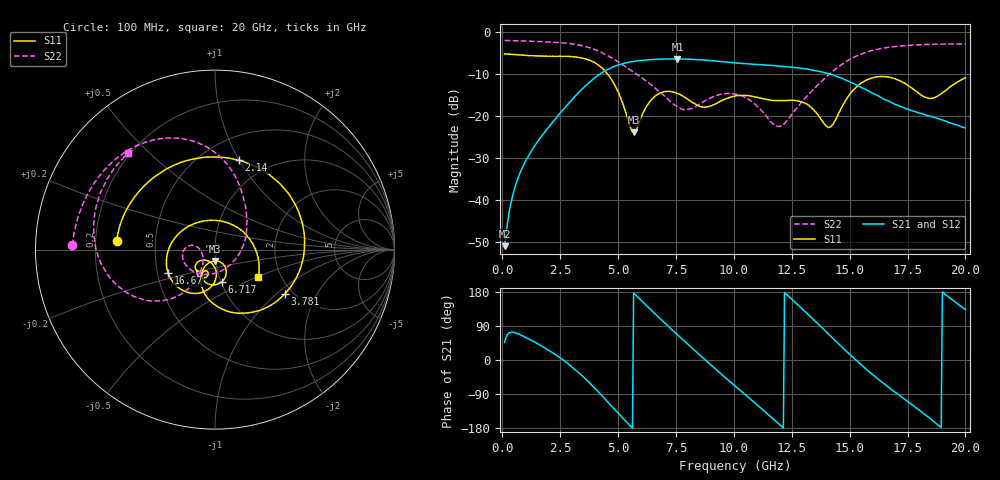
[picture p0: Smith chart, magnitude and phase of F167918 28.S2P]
!  2-Port S-parameters saved by WinCal
! VAR MeasName=S-Parameters (CALIBRATED_DATA) read from VNA (N5242A)
! VAR MeasDate=2016-11-22 10:26:05
! VAR NAME=F167918 28
! VAR FILENAME=F167918 28.S2P
! VAR DATE=2016-11-22 10:26:05
! VAR PHYS_PORTS=1,2
# Hz S DB R 50
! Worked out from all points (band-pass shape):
!   401 points, 100 MHz to 20 GHz, reference 50 ohm
!   highest |S21| = -6.38 dB at 7.562 GHz (marker M1); lowest = -50.9 dB at 100 MHz (marker M2)
!   |S21| within 3 dB of the highest: 4.385 GHz to 13.71 GHz (9.329 GHz wide, 103 % of centre)
!   lowest |S11| = -23.9 dB at 5.672 GHz (marker M3), VSWR 1.14, Z = 49.6 - j6.38 ohm
!   |S11| at or under -10 dB: 4.548 GHz to end of sweep
!   |S22| runs from -22.5 to -2.0 dB; largest |S21 - S12| = 0.0035
!   S11 on the Smith chart (normalised r, x): 100 MHz: 0.29, +0.04; 2.14 GHz: 0.74, +1.00; 3.781 GHz: 1.80, -1.14; 6.717 GHz: 1.01, -0.37; 16.67 GHz: 0.57, -0.16; 20 GHz: 1.53, -0.51
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1e8  -5.20 175.1  -50.91 46.7  -50.70 46.2  -2.00 178.3
7.4675e8  -5.44 144.4  -33.75 67.3  -33.68 67.2  -2.10 167.8
2.13975e9  -5.76 74.9  -21.67 20.4  -21.68 20.1  -2.39 144.2
2.886e9  -5.80 29.6  -16.79 -12.0  -16.80 -12.1  -2.73 129.2
3.43325e9  -6.17 -7.7  -13.63 -40.7  -13.63 -40.6  -3.23 116.4
3.7815e9  -6.74 -32.6  -11.86 -61.1  -11.84 -61.0  -3.75 107.6
4.7765e9  -11.83 -102.4  -8.31 -125.4  -8.28 -125.6  -6.32 82.2
5.672e9  -23.88 -89.6  -6.98 177.1  -6.97 176.9  -9.54 62.0
6.71675e9  -14.79 -77.7  -6.46 114.5  -6.46 114.7  -13.86 30.1
6.7665e9  -14.65 -79.7  -6.45 111.8  -6.45 111.8  -14.10 27.9
7.5625e9  -14.57 -108.3  -6.38 66.5  -6.39 66.5  -17.79 -20.5
8.7565e9  -17.87 -111.2  -6.68 0.3  -6.67 0.4  -16.34 -115.3
1.005e10  -15.21 -113.2  -7.31 -68.4  -7.29 -68.3  -14.74 -170.3
1.09455e10  -15.46 -126.2  -7.70 -115.1  -7.65 -115.2  -17.30 170.3
1.199025e10  -16.29 -128.7  -8.10 -171.2  -8.06 -171.4  -22.46 -156.7
1.338325e10  -18.17 -143.7  -9.01 109.9  -8.99 110.1  -13.94 -122.3
1.417925e10  -22.58 -110.6  -10.01 62.9  -10.04 63.1  -9.77 -128.4
1.53235e10  -12.91 -100.0  -12.65 -3.3  -12.62 -2.9  -5.62 -150.3
1.666675e10  -10.68 -153.2  -16.38 -71.3  -16.30 -71.1  -3.64 -178.5
1.67165e10  -10.76 -155.6  -16.48 -73.7  -16.47 -73.6  -3.62 -179.4
1.8408e10  -15.73 90.3  -19.94 -151.1  -19.86 -151.2  -2.94 153.2
2e10  -10.88 -32.3  -22.77 132.9  -22.62 133.5  -2.84 132.1
